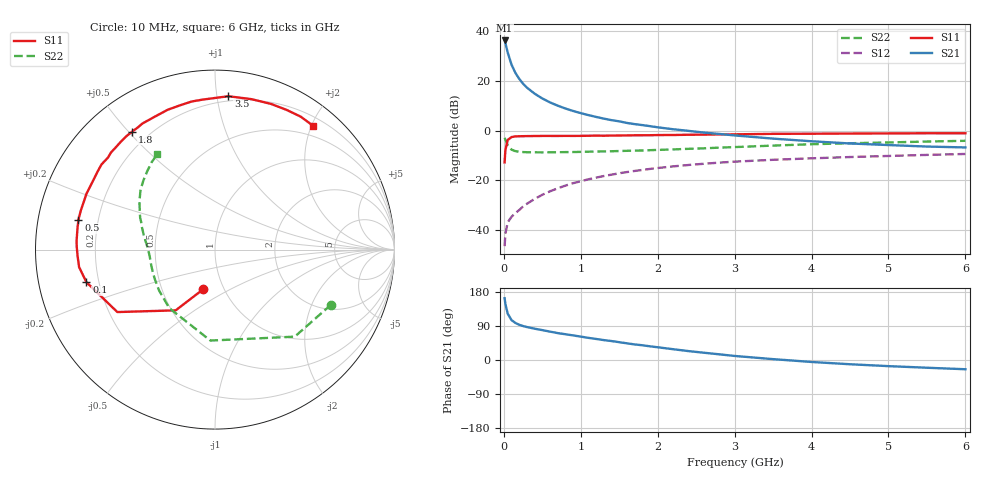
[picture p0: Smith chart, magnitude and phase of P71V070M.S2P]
! SIEMENS Small Signal Semiconductors
! BFP196
! Si NPN RF Bipolar Junction Transistor in SOT143
! VCE = 1 V  IC = 70 mA
! Common Emitter S-Parameters:  May  1996
# GHz  S  MA  R  50
!  f  S11  S21  S12  S22
! GHz  MAG  ANG  MAG  ANG  MAG  ANG  MAG  ANG
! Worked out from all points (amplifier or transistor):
!   36 points, 10 MHz to 6 GHz, reference 50 ohm
!   highest |S21| = 36.1 dB at 10 MHz (marker M1)
!   |S21| within 3 dB of that: start of sweep to 35.62 MHz
!   unconditionally stable (mu >= 1): 275.1 MHz to end of sweep
!   at 250 MHz: K = 0.97, MSG = 24.6 dB, |S12| = -30.5 dB
!   at 1.4 GHz: K = 1.13, MAG = 8.7 dB, |S12| = -17.7 dB
!   at 6 GHz: K = 1.03, MAG = 0.3 dB, |S12| = -9.4 dB
!   S11 on the Smith chart (normalised r, x): 10 MHz: 0.80, -0.37; 100 MHz: 0.15, -0.12; 500 MHz: 0.13, +0.11; 1.8 GHz: 0.14, +0.51; 3.5 GHz: 0.17, +1.08; 6 GHz: 0.33, +2.02
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0.01  0.2296 -106.4  63.93 163.0  0.0048 72.0  0.7156 -25.4
0.02  0.4031 -122.9  56.68 147.9  0.0085 62.4  0.6579 -47.5
0.05  0.6459 -147.4  36.8 122.2  0.0144 48.2  0.5074 -92.9
0.1  0.7392 -165.8  20.91 105.3  0.0186 46.4  0.4137 -128.0
0.15  0.7635 -172.7  14.32 97.8  0.0221 51.4  0.386 -143.8
0.2  0.7667 -177.6  10.86 92.9  0.0255 54.4  0.3746 -152.6
0.25  0.7704 178.9  8.669 89.6  0.03 57.3  0.3697 -158.7
0.3  0.7727 176.3  7.253 87.0  0.034 59.8  0.3672 -162.4
0.4  0.7753 171.2  5.482 82.6  0.0424 63.0  0.3655 -167.7
0.5  0.7789 167.7  4.39 78.9  0.0515 64.1  0.365 -171.3
0.6  0.7787 163.7  3.661 74.9  0.0604 64.4  0.3655 -173.8
0.7  0.7782 159.7  3.153 71.0  0.0693 64.1  0.3671 -175.7
0.9  0.7794 152.9  2.467 64.9  0.0878 62.6  0.3705 -179.1
1.1  0.7854 146.5  2.035 58.4  0.1052 60.3  0.3763 178.3
1.4  0.793 136.8  1.614 50.0  0.1304 56.1  0.3842 174.7
1.8  0.803 125.0  1.285 38.9  0.1621 49.7  0.3979 170.1
2.2  0.8131 114.3  1.061 28.5  0.1909 43.4  0.4176 165.0
2.8  0.8352 99.0  0.854 15.0  0.2269 34.0  0.4539 156.8
3.5  0.8578 85.0  0.688 2.3  0.2588 23.6  0.4987 147.6
4.5  0.8697 68.9  0.55 -11.2  0.2939 11.2  0.5555 135.8
5.5  0.8813 57.2  0.477 -20.4  0.3244 0.4  0.601 126.0
6  0.8801 51.7  0.458 -24.4  0.3386 -5.4  0.622 121.1
